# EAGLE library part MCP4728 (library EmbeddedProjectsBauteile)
MICROCHIP - MCP4728-E/UN - DAC 12BIT,QUAD,10MSOP
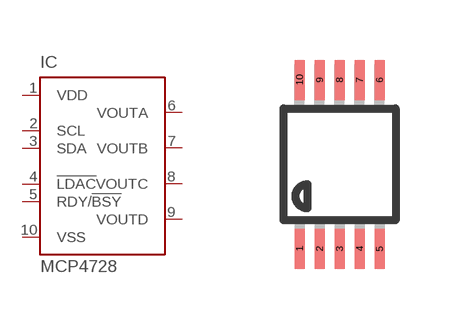
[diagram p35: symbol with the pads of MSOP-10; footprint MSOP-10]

Designator prefix IC

## MCP4728 (EP: 401108)  [MSOP-10]
1  VDD  pwr
2  SCL
3  SDA
4  !LDAC
5  RDY/!BSY  out
6  VOUTA  out
7  VOUTB  out
8  VOUTC  out
9  VOUTD  out
10  VSS  pwr

## Footprint MSOP-10 (pad centres in mm)
smd 0.25 x 1: 1 -1,-2.113; 2 -0.5,-2.113; 3 0,-2.113; 4 0.5,-2.113; 5 1,-2.113; 6 1,2.113; 7 0.5,2.113; 8 0,2.113; 9 -0.5,2.113; 10 -1,2.113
